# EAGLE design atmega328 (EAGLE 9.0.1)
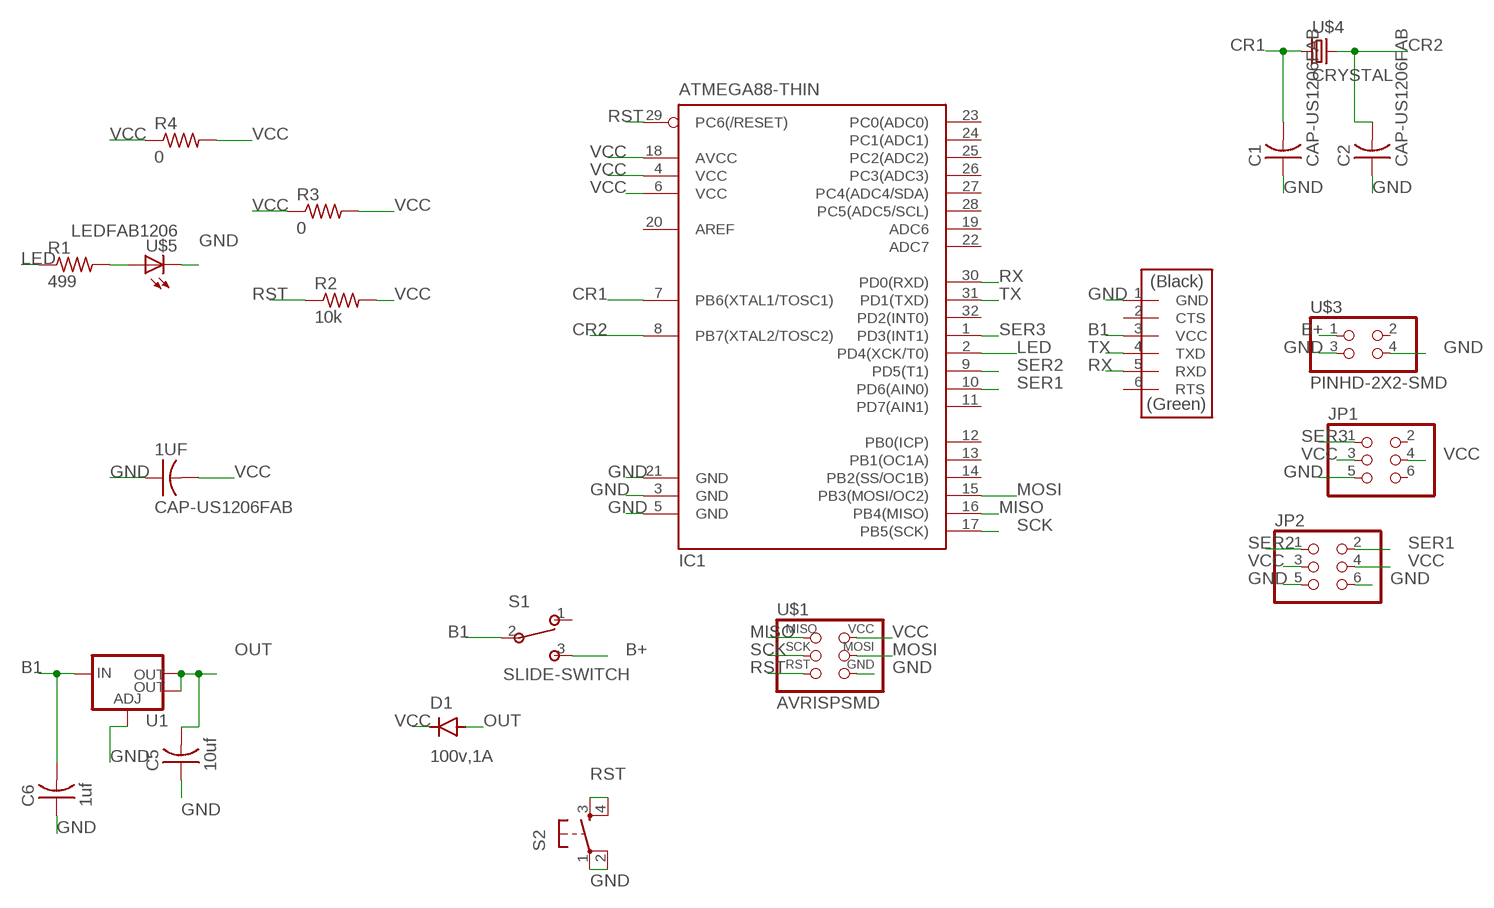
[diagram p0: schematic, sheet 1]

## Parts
1UF  CAP-US1206FAB  [C1206FAB]
C1  CAP-US1206FAB  [C1206FAB]
C2  CAP-US1206FAB  [C1206FAB]
C5  10uf  CAP-US1206FAB  [C1206FAB]
C6  1uf  CAP-US1206FAB  [C1206FAB]
D1  100v,1A  CDBM1100-G  [MINI-SMA]
IC1  ATMEGA88-THIN  [TQFP32-08THIN]
JP1  PINHD-2X3-SMD  [2X03SMD]
JP2  PINHD-2X3-SMD  [2X03SMD]
R1  499  RES-US1206FAB  [R1206FAB]
R2  10k  RES-US1206FAB  [R1206FAB]
R3  0  RES-US1206FAB  [R1206FAB]
R4  0  RES-US1206FAB  [R1206FAB]
S1  SLIDE-SWITCH  [AYZ0102AGRLC]
S2  6MM_SWITCH6MM_SWITCH  [6MM_SWITCH]
U1  V_REG_LM1117SOT223  [SOT223]
U$1  AVRISPSMD  [2X03SMD]
U$2  FTDI-SMD-HEADER  [1X06SMD]
U$3  PINHD-2X2-SMD  [2X02SMD]
U$4  CRYSTAL  [2-SMD-5X3MM]
U$5  LEDFAB1206  [LED1206FAB]

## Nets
B1: C6.2 S1.2 U1.3(IN) U$2.3(VCC)
B+: S1.3 U$3.1
CR1: C1.2 IC1.7(PB6(XTAL1/TOSC1)) U$4.P$1
CR2: C2.2 IC1.8(PB7(XTAL2/TOSC2)) U$4.P$2
GND: 1UF.1 C1.1 C2.1 C5.1 C6.1 IC1.3(GND) IC1.5(GND) IC1.21(GND) JP1.5 JP2.5 JP2.6 S2.1(P) S2.2(P1) U1.1(ADJ) U$1.6(GND) U$2.1(GND) U$3.3 U$3.4 U$5.2(C)
LED: IC1.2(PD4(XCK/T0)) R1.1
MISO: IC1.16(PB4(MISO)) U$1.1(MISO)
MOSI: IC1.15(PB3(MOSI/OC2)) U$1.4(MOSI)
N$2: R1.2 U$5.1(A)
OUT: C5.2 D1.ANODE U1.2(OUT) U1.4(OUT)
RST: IC1.29(PC6(/RESET)) R2.1 S2.3(S) S2.4(S1) U$1.5(RST)
RX: IC1.30(PD0(RXD)) U$2.5(RXD)
SCK: IC1.17(PB5(SCK)) U$1.3(SCK)
SER1: IC1.10(PD6(AIN0)) JP2.2
SER2: IC1.9(PD5(T1)) JP2.1
SER3: IC1.1(PD3(INT1)) JP1.1
TX: IC1.31(PD1(TXD)) U$2.4(TXD)
VCC: 1UF.2 D1.KATHODE IC1.4(VCC) IC1.6(VCC) IC1.18(AVCC) JP1.3 JP1.4 JP2.3 JP2.4 R2.2 R3.1 R3.2 R4.1 R4.2 U$1.2(VCC)
Unconnected: IC1.11(PD7(AIN1)) IC1.12(PB0(ICP)) IC1.13(PB1(OC1A)) IC1.14(PB2(SS/OC1B)) IC1.19(ADC6) IC1.20(AREF) IC1.22(ADC7) IC1.23(PC0(ADC0)) IC1.24(PC1(ADC1)) IC1.25(PC2(ADC2)) IC1.26(PC3(ADC3)) IC1.27(PC4(ADC4/SDA)) IC1.28(PC5(ADC5/SCL)) IC1.32(PD2(INT0)) JP1.2 JP1.6 S1.1 U$2.2(CTS) U$2.6(RTS) U$3.2

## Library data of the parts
1UF C1 C2 C5 C6 = fab:CAP-US
D1 = fab:CDBM1100-G: Diode schottky 100V 1A mini-SMA as found in the fablab inventory
IC1 = fab:ATMEGA88-THIN
JP1 JP2 = fab:PINHD-2X3-SMD: PIN HEADER
R1-R4 = fab:RES-US: Resistor (US Symbol)
S1 = fab:SLIDE-SWITCH: SMD slide-switch AYZ0102AGRLC as found in the fablab inventory. Includes the mounting holes. Made by Zaerc.
S2 = fab:6MM_SWITCH: OMRON SWITCH
U1 = fab:V_REG_LM1117: Voltage Regulator LM1117 Standard adjustable voltage regulator but in SMD form. Spark Fun Electronics SKU : COM-00595; PROD_ID: VREG-08170
U$1 = fab:AVRISP
U$2 = fab:FTDI-SMD-HEADER
U$3 = fab:PINHD-2X2-SMD
U$4 = fab:CRYSTAL
U$5 = fab:LED: LED

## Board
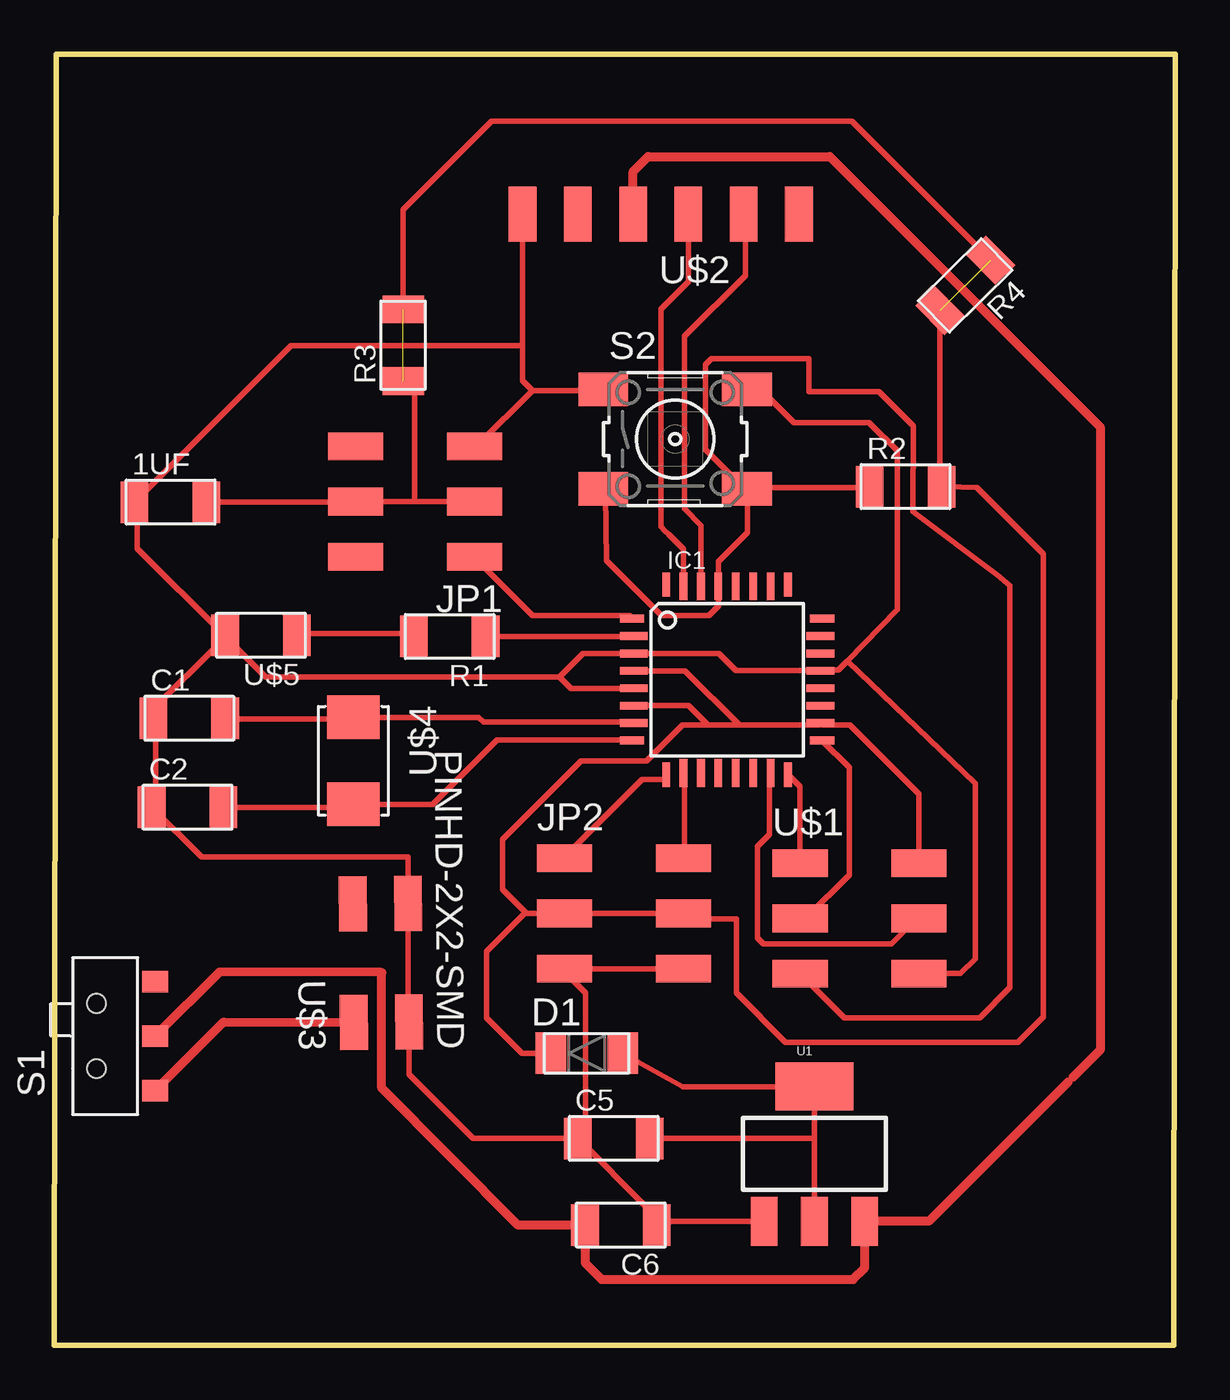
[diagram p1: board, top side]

Size 51.52 x 59.31 mm. Coordinates in mm from the lower left corner, seen from the top.
Outline: 0,0 51.44,0 51.52,59.31 0.08,59.31 0,0
Copper layers (1*16): Top 0.035mm / dielectric 1.5mm / Bottom 0.035mm
Design rules "default *": minimum track width 6mil, minimum drill 0.35mm, track to track 16mil, track to pad 16mil, pad to pad 16mil, via to via 16mil, smd to smd 16mil, copper to edge 40mil, drill to drill 6mil, minimum pad ring 10mil, minimum via ring 8mil, stop-mask expansion 4mil, vias tented up to drill 0mil, thermal gap 10mil

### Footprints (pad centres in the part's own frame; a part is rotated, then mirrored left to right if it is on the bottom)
C1206FAB = smd 1.27 x 1.905: 1 -1.651,0; 2 1.651,0
MINI-SMA = smd 1.4 x 1.9: ANODE 1.65,0; KATHODE -1.65,0
TQFP32-08THIN = smd 1.118 x 0.356: 1 -4.369,2.8; 8 -4.369,-2.8; 17 4.369,-2.8; 24 4.369,2.8 | smd 1.27 x 0.356: 2 -4.293,2; 3 -4.293,1.2; 4 -4.293,0.4; 5 -4.293,-0.4; 6 -4.293,-1.2; 7 -4.293,-2; 18 4.293,-2; 19 4.293,-1.2; 20 4.293,-0.4; 21 4.293,0.4; 22 4.293,1.2; 23 4.293,2 | smd 0.356 x 1.118: 9 -2.8,-4.369; 16 2.8,-4.369; 25 2.8,4.369; 32 -2.8,4.369 | smd 0.356 x 1.27: 10 -2,-4.293; 14 1.2,-4.293; 15 2,-4.293; 26 2,4.293; 27 1.2,4.293; 31 -2,4.293 | smd 0.35 x 1.27: 11 -1.2,-4.293; 12 -0.4,-4.293; 13 0.4,-4.293; 28 0.4,4.293; 29 -0.4,4.293; 30 -1.2,4.293
2X03SMD = smd 2.54 x 1.27: 1 -2.54,2.54; 2 2.92,2.54; 3 -2.54,0; 4 2.92,0; 5 -2.54,-2.54; 6 2.92,-2.54
R1206FAB = smd 1.27 x 1.905: 1 -1.651,0; 2 1.651,0
AYZ0102AGRLC = smd 1 x 1.2: 1 2.5,-2.3; 2 0,-2.3; 3 -2.5,-2.3 | hole 0.85: -1.5,0.4; 1.5,0.4
6MM_SWITCH = smd 2.286 x 1.524: 1 -3.302,2.286; 2 3.302,2.286; 3 -3.302,-2.286; 4 3.302,-2.286
SOT223 = smd 1.219 x 2.235: 1 -2.311,-3.099; 2 0,-3.099; 3 2.311,-3.099 | smd 3.6 x 2.2: 4 0,3.099
1X06SMD = smd 2.54 x 1.27: 1 0,6.35; 2 0,3.81; 3 0,1.27; 4 0,-1.27; 5 0,-3.81; 6 0,-6.35
2X02SMD = smd 2.54 x 1.27: 1 -2.54,1.27; 2 2.92,1.27; 3 -2.54,-1.27; 4 2.92,-1.27
2-SMD-5X3MM = smd 2 x 2.4: P$1 -2,0; P$2 2,0
LED1206FAB = smd 1.27 x 1.905: 1 -1.651,0; 2 1.651,0

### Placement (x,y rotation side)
1UF  5.33,38.73 0 top
C1  6.2,28.8 0 top
C2  6.12,24.71 0 top
C5  25.7,9.5 0 top
C6  26.03,5.51 180 top
D1  24.46,13.41 0 top
IC1  30.91,30.58 0 top
JP1  16.76,38.76 180 top
JP2  25.98,19.84 0 top
R1  18.16,32.56 180 top
R2  39.12,39.45 0 top
R3  16.03,45.95 90 top
R4  41.86,48.69 224.7 top
S1  2.34,14.2 90 top
S2  28.52,41.63 0 top
U1  34.92,8.79 0 top
U$1  36.8,19.61 0 top
U$2  27.86,51.97 90 top
U$3  15.01,17.37 90.5 top
U$4  13.74,26.85 270 top
U$5  9.5,32.61 180 top

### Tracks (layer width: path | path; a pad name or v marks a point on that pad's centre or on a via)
B1
  Top 0.152: 23.82,5.56 C6.2 | 26.44,51.97 U$2.3 26.72,51.97
  Top 0.254: 46.58,12.09 46.81,12.32 | U$2.3 26.59,52.98
  Top 0.406: S1.2 7.58,17.14 15.04,17.12 15.04,11.81 21.31,5.51 C6.2 24.38,3.78 25.15,3.02 36.7,3.02 37.24,3.56 U1.3 40.18,5.69 46.58,12.09 | U$2.3 26.59,53.92 27.28,54.61 35.64,54.61 48.06,42.19 48.06,13.56 46.81,12.32
B+
  Top 0.406: S1.3 7.79,14.85 U$3.1
CR1
  Top 0.152: 14.15,28.5 13.87,28.78 U$4.P$1 13.59,28.78 | 8,28.78 C1.2
  Top 0.254: 13.59,28.78 8,28.78 | U$4.P$1 19.49,28.85 19.71,28.63 26.57,28.63 IC1.7
CR2
  Top 0.152: 8,24.87 C2.2
  Top 0.254: IC1.8 26.51,27.81 20.35,27.81 17.38,24.85 U$4.P$2 13.61,24.71 C2.2
GND
  Top 0.152: 27.18,5.28 27.26,5.47 | 27.26,5.47 C6.1 27.46,5.56 | 35.1,31.01 IC1.21 35.38,31.01 | 32.03,43.87 S2.2 | 39.85,17.32 U$1.6 40.69,17.07 | 25.04,43.87 S2.1 | 19.46,41.35 JP1.5 19.18,41.07 | 4.65,24.87 C2.1 4.37,24.59 | 4.65,28.78 C1.1 4.37,29.06 | 7.72,32.41 U$5.2 | 3.81,38.56 1UF.1 3.81,38.84 | 7.72,32.69 U$5.2 | U$5.2 8,32.41 | 27.48,5.69 27.26,5.47 | C5.1 24.41,9.86 | 27.26,6.29 27.26,5.47 | 19.23,9.5 19.21,9.5 | U$3.4 16.26,20.24 | 16.26,20.24
  Top 0.254: 21.97,43.87 25.04,43.87 | 19.46,41.35 21.97,43.87 | 4.65,28.78 4.65,24.87 | 4.37,29.06 7.72,32.41 | 3.81,38.56 3.81,36.6 7.72,32.69 | U1.1 27.48,5.69 | 24.41,9.86 24.41,16.19 23.44,17.16 JP2.5 JP2.6 | 27.26,6.29 C5.1 19.23,9.5 16.29,12.43 U$3.3 16.26,14.89 U$3.4 | C2.1 6.76,22.43 16.26,22.43 16.26,20.24 | 36.44,31.43 38.73,33.81 38.73,41.1 37.44,42.39 33.98,42.39 32.49,43.89 31.8,43.89 S2.2 | 36.44,31.43 36.02,31.01 35.38,31.01 | 36.44,31.43 42.32,25.81 42.32,17.75 41.63,17.07 U$1.6 | IC1.21 31.32,30.99 30.53,31.78 IC1.3 24.29,31.78 23.22,30.71 | S2.1 25.22,44.3 | 1UF.1 10.87,45.92 21.51,45.92 | 21.51,45.92 U$2.1 | 23.22,30.71 9.7,30.71 8,32.41 | IC1.5 23.74,30.18 23.22,30.71 | 21.51,45.92 21.51,44.32 21.97,43.87
LED
  Top 0.152: 20.01,32.66 R1.1
  Top 0.254: R1.1 26.6,32.56 IC1.2
MISO
  Top 0.152: 34.29,22.35 U$1.1
  Top 0.254: U$1.1 34.26,25.66 IC1.16
MOSI
  Top 0.152: 32.87,26.26 IC1.15 | 39.57,19.56 U$1.4
  Top 0.254: 32.87,26.26 32.87,23.47 32.31,22.91 32.31,18.72 32.59,18.44 38.46,18.44 39.57,19.56
N$2
  Top 0.152: 16.38,32.69 R1.2 | 11.35,32.69 U$5.1
  Top 0.254: 11.35,32.69 16.38,32.69
OUT
  Top 0.152: 34.92,11.86 U1.4 | 34.9,9.5 34.92,9.47
  Top 0.254: U1.2 34.92,9.47 34.92,11.86 30.84,11.86 28.88,11.86 D1.ANODE | C5.2 34.9,9.5
RST
  Top 0.152: 37.34,39.4 R2.1 | 32.03,39.4 S2.4 31.6,39.47 | 25.32,39.12 S2.3 | 34.26,17.04 U$1.5
  Top 0.254: 32.03,39.4 37.34,39.4 | 25.32,39.12 25.37,36.04 27.89,33.53 30.07,33.53 30.51,33.97 IC1.29 30.51,36 31.85,37.34 31.85,39.32 S2.4 | 31.6,39.47 29.92,41.15 29.92,45.06 30.2,45.34 34.67,45.34 34.67,43.81 37.9,43.81 39.47,42.24 39.45,38.3 43.33,35.38 43.92,34.9 43.92,16.43 42.52,15.04 36.3,15.04 U$1.5
RX
  Top 0.152: 31.75,51.97 U$2.5
  Top 0.254: 31.75,51.97 31.75,49.15 28.96,46.35 28.96,38.43 29.72,37.67 IC1.30
SCK
  Top 0.152: 35.38,27.66 IC1.17 | 34.57,19.66 U$1.3
  Top 0.254: 34.57,19.66 36.52,21.62 36.52,26.54 IC1.17
SER1
  Top 0.152: 28.96,26.26 IC1.10 | 28.96,22.63 JP2.2
  Top 0.254: 28.96,22.63 28.96,26.26
SER2
  Top 0.152: 28.12,25.98 IC1.9 | 23.65,22.63 JP2.1
  Top 0.254: 28.12,25.98 27,25.98 23.65,22.63
SER3
  Top 0.152: 26.44,33.53 IC1.1 | 19.46,36.04 JP1.1
  Top 0.254: 26.44,33.53 21.97,33.53 19.46,36.04
TX
  Top 0.152: 28.96,34.92 IC1.31
  Top 0.254: IC1.31 28.91,36.57 28.22,37.26 28.07,37.41 27.86,37.62 27.86,47.6 29.13,48.87 U$2.4
VCC  (2 unrouted)
  Top 0.152: 23.37,19.84 JP2.3 | 26.72,31.01 IC1.4 | 39.57,22.35 U$1.2 | 19.18,38.56 JP1.3 19.42,38.82 19.46,38.84 | 21.62,19.84 21.69,19.84
  Top 0.254: 28.88,19.84 JP2.3 21.69,19.84 20.6,20.93 20.6,23.24 24.21,26.85 27.2,26.85 28.85,28.5 30.02,28.5 | 28.88,19.84 JP2.4 | 40.97,39.44 42.39,39.4 45.44,36.35 45.44,15.09 44.27,13.92 33.6,13.92 31.34,16.18 31.34,19.58 29.13,19.58 28.88,19.84 | 40.97,39.44 R2.2 | D1.KATHODE 21.49,13.41 19.86,15.04 19.86,18.08 21.62,19.84 | U$1.2 39.72,25.32 36.55,28.5 35.29,28.5 IC1.18 35.12,28.5 31.47,28.5 | JP1.4 13.79,38.71 | JP1.4 16.56,38.76 | 16.56,38.76 19.36,38.76 19.42,38.82 | 16.56,38.76 16.56,43.76 R3.1 | R4.2 40.69,39.72 40.97,39.44 | R4.1 36.65,56.24 20.09,56.24 16.03,52.17 R3.2 | 1UF.2 13.82,38.73 JP1.4 | 30.02,28.5 31.34,28.5 31.47,28.5 | IC1.6 29.14,29.38 30.02,28.5 | IC1.4 28.99,30.98 31.47,28.5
